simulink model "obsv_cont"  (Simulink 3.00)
settings: Solver=ode45  StartTime=0.0  StopTime=10.0  RelTol=1e-3
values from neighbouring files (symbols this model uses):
  A = [a11 a12 0 -g;a21 a22 1 0;a31 a31 a33 0;0 1 0 0]    [EXP7_3.M]    (also in EXP6_10.M = [0 1 0;0 -1.799 6.953;0 0.939 -1.660]; EXP6_8.M; EXP6_9.m; EXP7_1.M = [0 1 0 0;0 0 -mb*g/(1-mb) 0;0 0 0 1;0 0 m2_bar*g/(1-mb) 0])
  B = [b1;b2;b3;0]    [EXP7_3.M]    (also in EXP6_10.M = [0 0;-28.97 -6.453;-0.174 -0.230]; EXP6_8.M; EXP6_9.m; EXP7_1.M = [0;1/((m+M)*(1-mb));0;-m2_bar/((m+M)*(1-mb))])
  C = [1 0 0 0]    [EXP7_3.M]    (also in EXP6_8.M; EXP6_9.m; EXP7_1.M; EXP7_2.M = [1 0 0 0;0 0 1 0])
  K = acker(A,B,Pc)    [EXP7_3.M]    (also in EXP6_10.M = Q*inv(V); EXP6_8.M = acker(A,B,P); EXP6_9.m = acker(A_bar,B_bar,P); Exp7_4.m = [0.922 -6.5955 -2.35 -8.977])
  L = (acker(A',C',Po))'    [EXP7_3.M]    (also in EXP5_3.M = 0.35; ODE.M = par_in(5); EXP7_1.M = L_ext'; EXP7_2.M = [-10 1 0 0;0 0 -10 1])
libraries: simulink3 x8

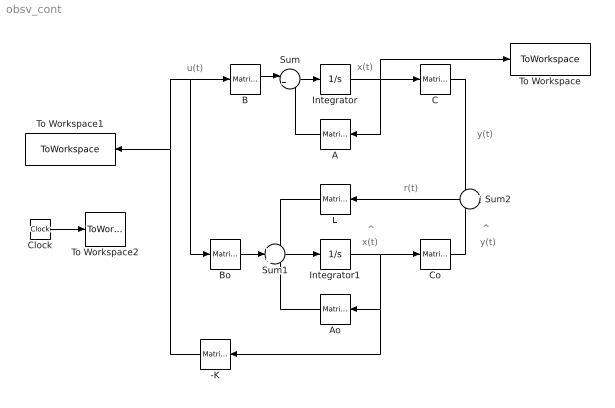
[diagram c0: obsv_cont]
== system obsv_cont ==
  note: u(t)
  note: x(t)
  note: r(t)
  note: y(t)
  note: y(t)
  note: ^
  note: x(t)
  note: ^
  -K : simulink3/Math/Matrix Gain  Orientation=left  K=-K
  A : simulink3/Math/Matrix Gain  Orientation=left  K=A
  Ao : simulink3/Math/Matrix Gain  Orientation=left  K=A
  B : simulink3/Math/Matrix Gain  K=B
  Bo : simulink3/Math/Matrix Gain  K=B
  C : simulink3/Math/Matrix Gain  K=C
  Clock : Clock
  Co : simulink3/Math/Matrix Gain  K=C
  Integrator : Integrator  ExternalReset=none  InitialConditionSource=internal  InitialCondition=[0.2 .1 -0.5 0.5]  LimitOutput=off  UpperSaturationLimit=inf  LowerSaturationLimit=-inf  ShowSaturationPort=off  ShowStatePort=off  AbsoluteTolerance=auto
  Integrator1 : Integrator  ExternalReset=none  InitialConditionSource=internal  InitialCondition=0  LimitOutput=off  UpperSaturationLimit=inf  LowerSaturationLimit=-inf  ShowSaturationPort=off  ShowStatePort=off  AbsoluteTolerance=auto
  L : simulink3/Math/Matrix Gain  Orientation=left  K=L
  Sum : Sum  Inputs=|++  SaturateOnIntegerOverflow=on
  Sum1 : Sum  Inputs=+++  SaturateOnIntegerOverflow=on
  Sum2 : Sum  Orientation=left  Inputs=+-  SaturateOnIntegerOverflow=on
  To Workspace : ToWorkspace  VariableName=obsv_cont_states  SampleTime=-1  SaveFormat=Matrix
  To Workspace1 : ToWorkspace  VariableName=obsv_cont_control  SampleTime=-1  SaveFormat=Matrix
  To Workspace2 : ToWorkspace  VariableName=time2  SampleTime=-1  SaveFormat=Matrix
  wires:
  B/1 -> Sum/1
  Sum/1 -> Integrator/1
  Integrator/1 -> C/1, A/1, To Workspace/1
  Sum1/1 -> Integrator1/1
  C/1 -> Sum2/1
  Co/1 -> Sum2/2
  Bo/1 -> Sum1/2
  Integrator1/1 -> Co/1, Ao/1, -K/1
  L/1 -> Sum1/1
  A/1 -> Sum/2
  Ao/1 -> Sum1/3
  Sum2/1 -> L/1
  -K/1 -> B/1, Bo/1, To Workspace1/1
  Clock/1 -> To Workspace2/1
